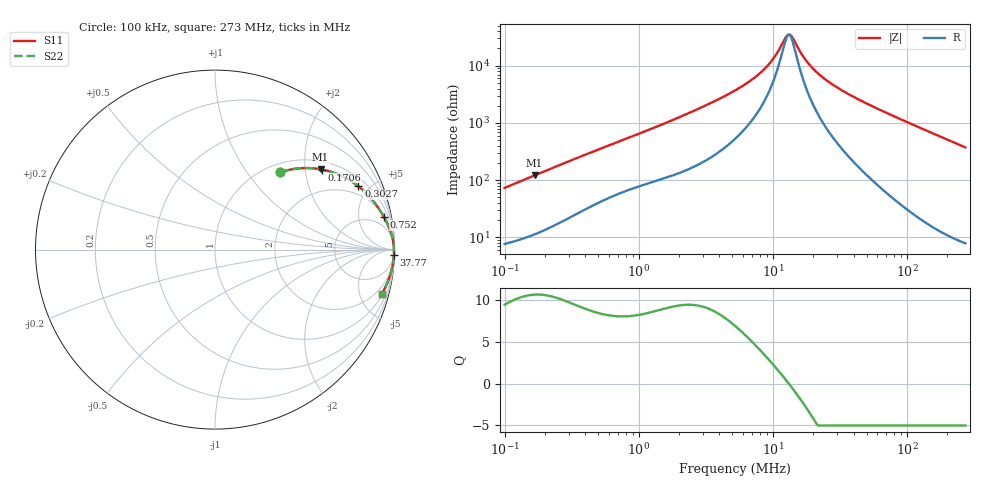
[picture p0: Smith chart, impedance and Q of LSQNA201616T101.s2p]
! LSQNA201616T101  S-PARAMETER MODEL  ( General Type )
! Model Generated by TAIYO YUDEN Corporation (http://www.ty-top.com)
! Version 2.0
! TAIYO YUDEN Control No. 100810NF25SB-FKC
! Copyright(c) 2007 TAIYO YUDEN CO.,LTD. All Rights Reserved.
! Product Description (link to TY-COMPAS)
! https://ds.yuden.co.jp/TYCOMPAS/or/detail?pn=LSQNA201616T101K&u=M
! Products Name : Inductors
! Characteristics :
!  Inductance : 100 uH , SRF(min) : 8.0 MHz , DC Resistance(max) : 5.85 Ohm
!  Rated Current : Saturation :70 mA , Temp Rise : 170 mA (40 degC)
!  Case Size : 2.0 x 1.6 / 0.079 x 0.063 [mm/inch] , Thickness : 1.6 / 0.063 [mm/inch]
!  (Conditions: Temperature = 25 degC , DC Bias Current/Voltage = 0A / 0V)
! External Node Assignments :
!  1  o---GGG---o  2
! GND o---------o GND
! Frequency Range : 0.1MHz  -  272.98108MHz  [ 402 STEP ]
# MHz S RI R 50
! Freq[MHz].  S11 Real  S11 Imag  S21 Real  S21 Imag  S12 Real  S12 Imag  S22 Real  S22 Imag
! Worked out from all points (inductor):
!   401 points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, 100 kHz to 273 MHz, reference 50 ohm
!   read as one part in series: L = 116 uH near 104 kHz
!   highest Q = 10.7 at 167.2 kHz (marker M1), where L = 115 uH
!   self-resonance near 12.98 MHz
!   S11 on the Smith chart (normalised r, x): 100 kHz: 1.15, +1.46; 170.6 kHz: 1.23, +2.47; 302.7 kHz: 1.44, +4.28; 752 kHz: 2, +10; 37.77 MHz: 6, -61; 273 MHz: 1.16, -7.49
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0.1  0.3645 0.4314  0.6355 -0.4314  0.6355 -0.4314  0.3645 0.4314
0.167243  0.5882 0.4476  0.4118 -0.4476  0.4118 -0.4476  0.5882 0.4476
0.170584  0.5967 0.446  0.4033 -0.446  0.4033 -0.446  0.5967 0.446
0.302732  0.7992 0.3526  0.2008 -0.3526  0.2008 -0.3526  0.7992 0.3526
0.376316  0.8496 0.307  0.1504 -0.307  0.1504 -0.307  0.8496 0.307
0.751993  0.9404 0.1829  0.0596 -0.1829  0.0596 -0.1829  0.9404 0.1829
1.416134  0.9759 0.1069  0.0241 -0.1069  0.0241 -0.1069  0.9759 0.1069
3.062861  0.992 0.0501  0.00802 -0.0501  0.00802 -0.0501  0.992 0.0501
5.329134  0.9955 0.0259  0.00448 -0.0259  0.00448 -0.0259  0.9955 0.0259
7.169875  0.9964 0.0163  0.00362 -0.0163  0.00362 -0.0163  0.9964 0.0163
8.912617  0.9968 0.0101  0.00323 -0.0101  0.00323 -0.0101  0.9968 0.0101
10.23617  0.9969 0.00647  0.00305 -0.00647  0.00305 -0.00647  0.9969 0.00647
12.23068  0.9971 0.0019  0.00289 -0.0019  0.00289 -0.0019  0.9971 0.0019
12.97841  0.9972 0.000396  0.00285 -0.000396  0.00285 -0.000396  0.9972 0.000396
14.04698  0.9972 -0.00162  0.0028 0.00162  0.0028 0.00162  0.9972 -0.00162
16.78401  0.9972 -0.00622  0.00275 0.00622  0.00275 0.00622  0.9972 -0.00622
19.66158  0.9972 -0.0105  0.00277 0.0105  0.00277 0.0105  0.9972 -0.0105
25.93481  0.9971 -0.0187  0.00293 0.0187  0.00293 0.0187  0.9971 -0.0187
37.76586  0.9964 -0.0322  0.00359 0.0322  0.00359 0.0322  0.9964 -0.0322
73.9896  0.9925 -0.0695  0.00753 0.0695  0.00753 0.0695  0.9925 -0.0695
144.9579  0.9774 -0.1372  0.0226 0.1372  0.0226 0.1372  0.9774 -0.1372
272.9811  0.929 -0.2465  0.071 0.2465  0.071 0.2465  0.929 -0.2465
